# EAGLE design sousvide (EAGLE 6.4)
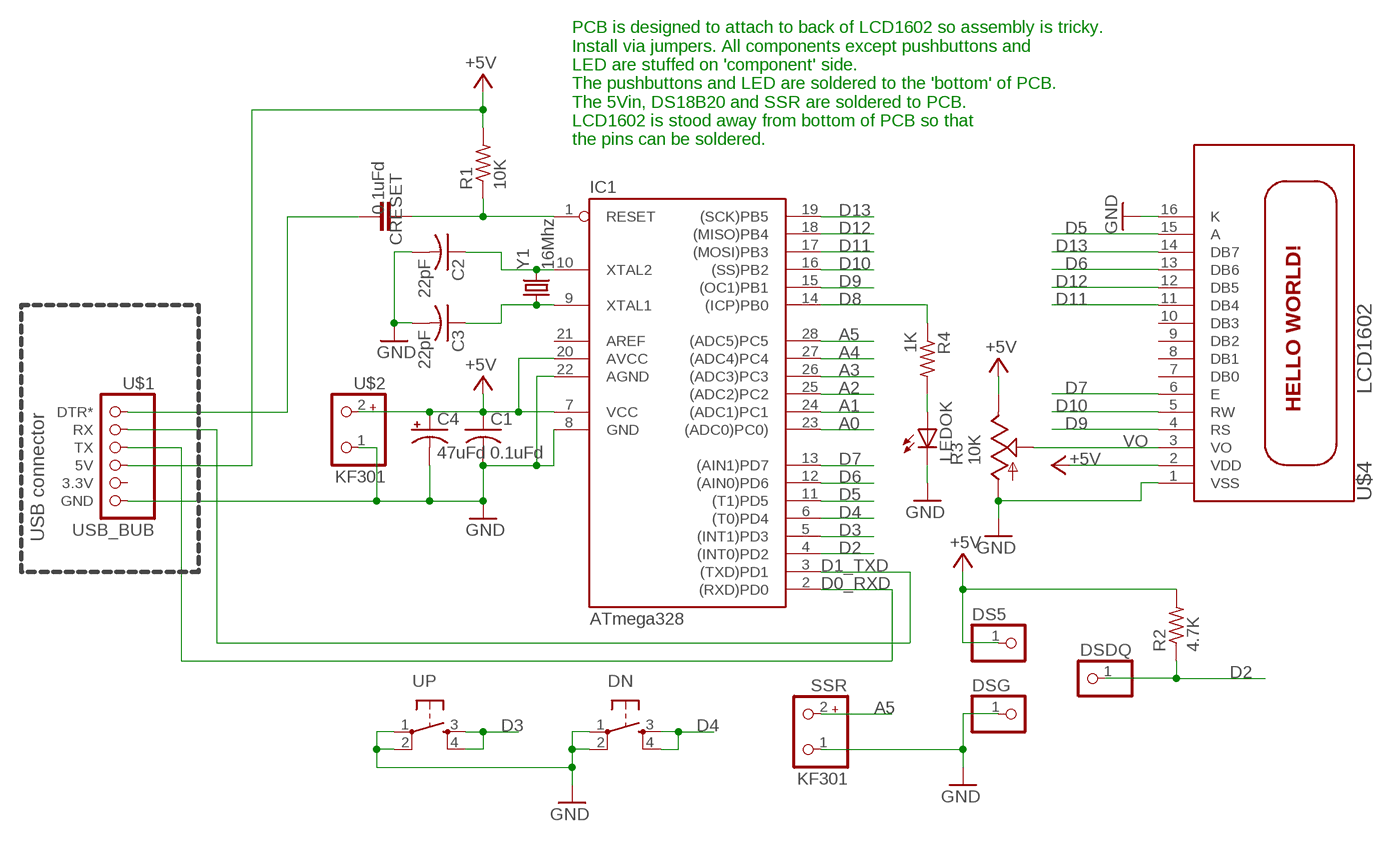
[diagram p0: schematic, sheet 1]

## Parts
C1  0.1uFd  C-US050-024X044  [C050-024X044]
C2  22pF  C-US025-024X044  [C025-024X044]
C3  22pF  C-US025-024X044  [C025-024X044]
C4  47uFd  CPOL-USE5-8.5  [E5-8,5]
CRESET  0.1uFd  C-EU050-045X075  [C050-045X075]
DN  TAC_SWITCHPTH  [TACTILE-PTH]
DS5  PINHD-1X1  [1X01]
DSDQ  PINHD-1X1  [1X01]
DSG  PINHD-1X1  [1X01]
IC1  ATmega328  AT90S4433P  [DIL28-3]
LEDOK  LED5MM  [LED5MM]
R1  10K  R-US_0207/2V  [0207/2V]
R2  4.7K  R-US_0204/7  [0204/7]
R3  10K  TRIM_US-B64Y  [B64Y]
R4  1K  R-US_0207/7  [0207/7]
SSR  KF301  [KF301]
U$1  USB_BUB  [USB_BUB]
U$2  KF301  [KF301]
U$4  LCD1602  [LCD1602]
UP  TAC_SWITCHPTH  [TACTILE-PTH]
Y1  16Mhz  CRYSTALHC49US  [HC49US]

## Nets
+5V [power]: C1.1 C4.+ DS5.1 IC1.7(VCC) IC1.20(AVCC) R1.2 R2.2 R3.E U$1.5V U$2.2 U$4.2(VDD)
A0: IC1.23((ADC0)PC0))
A1: IC1.24((ADC1)PC1)
A2: IC1.25((ADC2)PC2)
A3: IC1.26((ADC3)PC3)
A4: IC1.27((ADC4)PC4)
A5: IC1.28((ADC5)PC5) SSR.2
D0_RXD: IC1.2((RXD)PD0) U$1.TX
D1_TXD: IC1.3((TXD)PD1) U$1.RX
D2: DSDQ.1 IC1.4((INT0)PD2) R2.1
D3: IC1.5((INT1)PD3) UP.3 UP.4
D4: DN.3 DN.4 IC1.6((T0)PD4)
D5: IC1.11((T1)PD5) U$4.15(A)
D6: IC1.12((AIN0)PD6) U$4.13(DB6)
D7: IC1.13((AIN1)PD7) U$4.6(E)
D8: IC1.14((ICP)PB0) R4.1
D9: IC1.15((OC1)PB1) U$4.4(RS)
D10: IC1.16((SS)PB2) U$4.5(RW)
D11: IC1.17((MOSI)PB3) U$4.11(DB4)
D12: IC1.18((MISO)PB4) U$4.12(DB5)
D13: IC1.19((SCK)PB5) U$4.14(DB7)
GND [power]: C1.2 C2.2 C3.2 C4.- DN.1 DN.2 DSG.1 IC1.8(GND) IC1.22(AGND) LEDOK.K(C) R3.A SSR.1 U$1.GND U$2.1 U$4.1(VSS) U$4.16(K) UP.1 UP.2
N$1: LEDOK.A R4.2
N$6: C3.1 IC1.9(XTAL1) Y1.1
N$7: C2.1 IC1.10(XTAL2) Y1.2
N$8: CRESET.1 U$1.DTR*
RESET: CRESET.2 IC1.1(RESET) R1.1
VO: R3.S U$4.3(VO)
Unconnected: IC1.21(AREF) U$1.3.3V U$4.7(DB0) U$4.8(DB1) U$4.9(DB2) U$4.10(DB3)

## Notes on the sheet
- PCB is designed to attach to back of LCD1602 so assembly is tricky.
  Install via jumpers. All components except pushbuttons and
  LED are stuffed on 'component' side.
  The pushbuttons and LED are soldered to the 'bottom' of PCB. 
  The 5Vin, DS18B20 and SSR are soldered to PCB.
  LCD1602 is stood away from bottom of PCB so that
  the pins can be soldered.
- USB connector

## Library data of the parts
C1-C3 = MTS:C-US: CAPACITOR, American symbol
C4 = rcl:CPOL-US: POLARIZED CAPACITOR, American symbol
CRESET = my-rcl:C-EU: CAPACITOR, European symbol
DN UP = SparkFun:TAC_SWITCH: Momentary Switch Button commonly used for reset or general input. Spark Fun Electronics SKU : COM-00097
DS5 DSDQ DSG = pinhead:PINHD-1X1: PIN HEADER
IC1 = atmel:AT90S4433: MICROCONTROLLER 4 Kbytes FLASH 128 bytes SRAM 256 bytes EEPROM UART 6-channel 10 bit ADC
LEDOK = SparkFun:LED: LEDs
R1 R2 R4 = MTS:R-US_: RESISTOR, American symbol
R3 = pot:TRIM_US-: POTENTIOMETER
SSR U$2 = MTS_Custom:KF301
U$1 = MTS:USB_BUB
U$4 = MTS_Custom:LCD1602
Y1 = MTS:CRYSTAL: Crystals

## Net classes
0 default: width 0.4 mm, clearance 0.3 mm
1 power: width 0.6 mm, clearance 0.3 mm

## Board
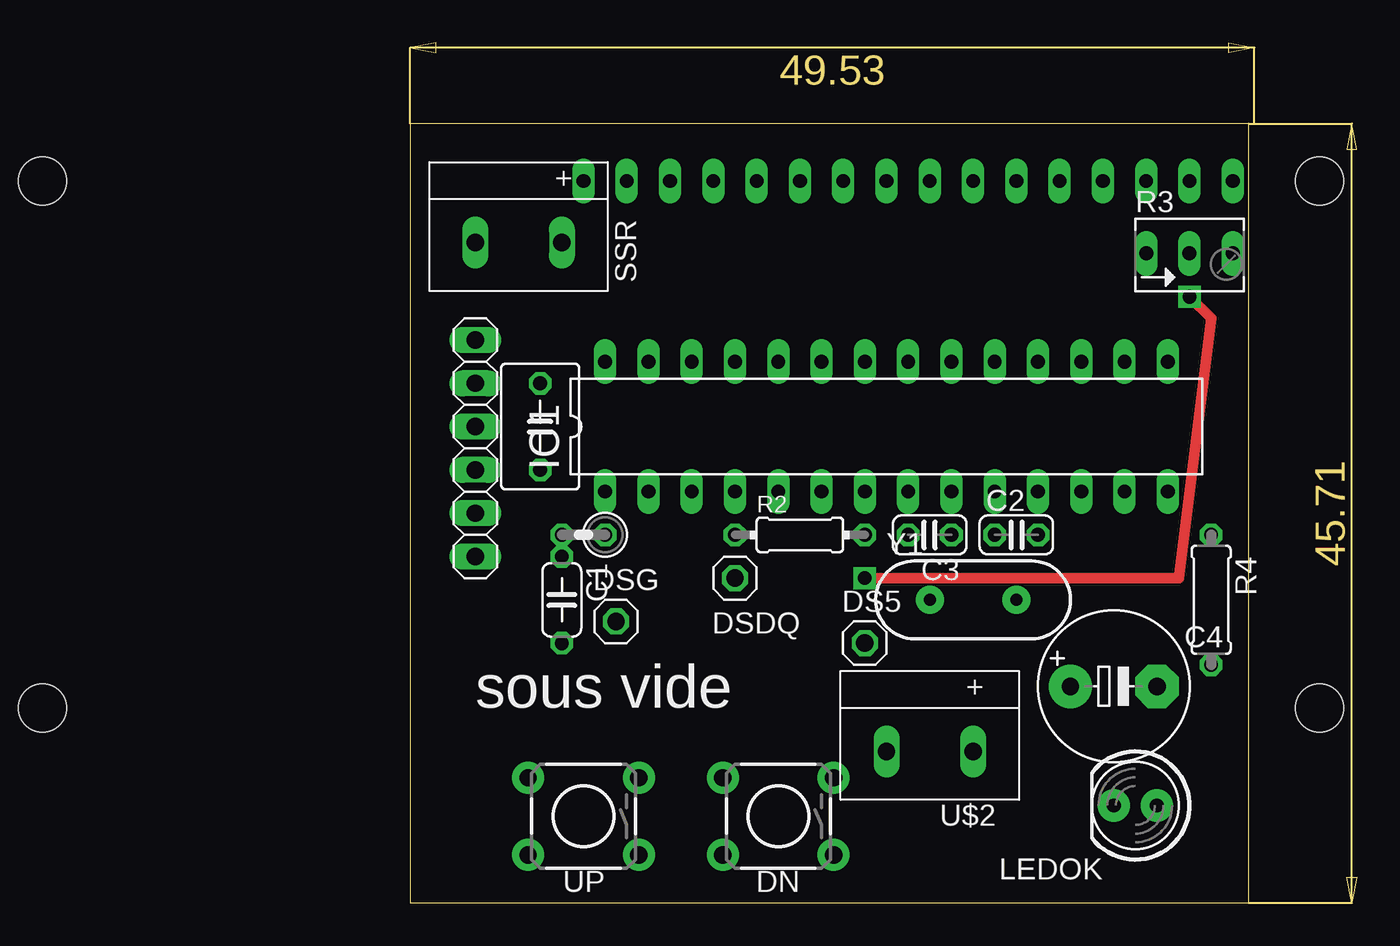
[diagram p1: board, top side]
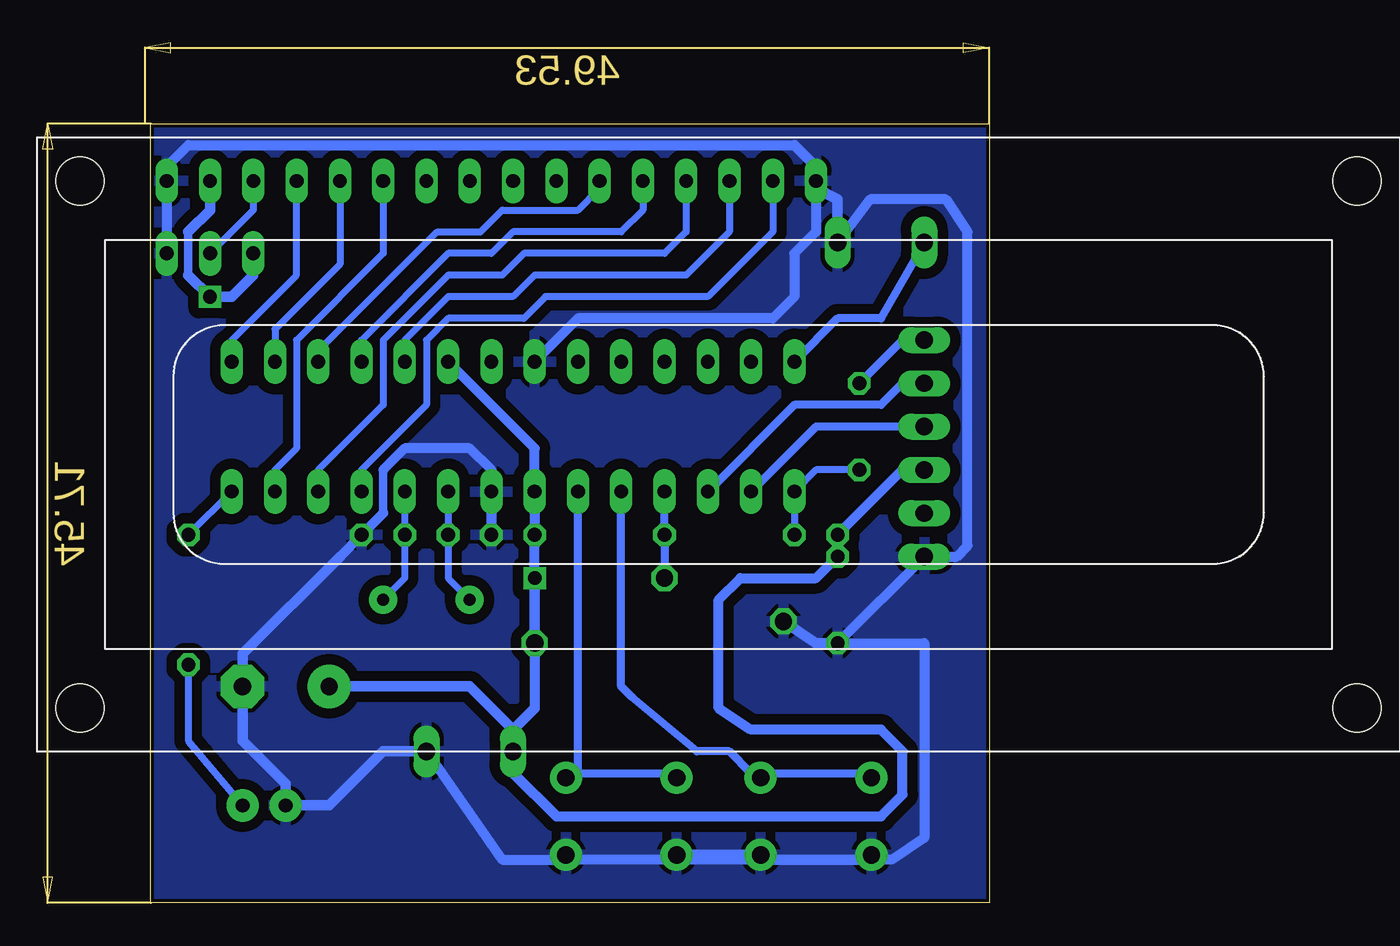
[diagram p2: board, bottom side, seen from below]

Size 55.54 x 50.46 mm. Coordinates in mm from the lower left corner, seen from the top.
Outline: 0,0 49.2,0 49.2,45.71 0,45.71 0,0
Copper layers (1*16): Top 0.035mm / dielectric 1.5mm / Bottom 0.035mm
Design rules "MTS": minimum track width 18mil, minimum drill 12mil, track to track 24mil, track to pad 24mil, pad to pad 6mil, via to via 6mil, smd to smd 0mil, copper to edge 8mil, drill to drill 10mil, minimum pad ring 10mil, minimum via ring 10mil, stop-mask expansion 2mil, vias tented up to drill 25mil, thermal gap 10mil

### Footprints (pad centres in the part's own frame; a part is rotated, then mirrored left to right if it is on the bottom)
C050-024X044 = drill 0.813 octagon: 1 -2.54,0; 2 2.54,0
C025-024X044 = drill 0.813 octagon: 1 -1.27,0; 2 1.27,0
E5-8,5 = drill 1.016 pad 2.54: + -2.54,0 | drill 1.016 pad 2.54 octagon: - 2.54,0
C050-045X075 = drill 0.813 octagon: 1 -2.54,0; 2 2.54,0
TACTILE-PTH = drill 1.016 pad 1.88: 1 -3.251,2.261; 2 3.251,2.261; 3 -3.251,-2.261; 4 3.251,-2.261
1X01 = drill 1.016 octagon: 1 0,0
DIL28-3 = drill 0.813 long: 1 -16.51,-3.81; 2 -13.97,-3.81; 3 -11.43,-3.81; 4 -8.89,-3.81; 5 -6.35,-3.81; 6 -3.81,-3.81; 7 -1.27,-3.81; 8 1.27,-3.81; 9 3.81,-3.81; 10 6.35,-3.81; 11 8.89,-3.81; 12 11.43,-3.81; 13 13.97,-3.81; 14 16.51,-3.81; 15 16.51,3.81; 16 13.97,3.81; 17 11.43,3.81; 18 8.89,3.81; 19 6.35,3.81; 20 3.81,3.81; 21 1.27,3.81; 22 -1.27,3.81; 23 -3.81,3.81; 24 -6.35,3.81; 25 -8.89,3.81; 26 -11.43,3.81; 27 -13.97,3.81; 28 -16.51,3.81
LED5MM = drill 0.813 pad 1.88: A -1.27,0; K 1.27,0
0207/2V = drill 0.813 octagon: 1 -1.27,0; 2 1.27,0
0204/7 = drill 0.813 octagon: 1 -3.81,0; 2 3.81,0
B64Y = drill 0.813 long: A 2.54,0; E -2.54,0; S 0,0
0207/7 = drill 0.813 octagon: 1 -3.81,0; 2 3.81,0
KF301 = drill 1.016 long: 1 -2.54,0; 2 2.54,0
USB_BUB = drill 1.016 long: 3.3V -3.81,0; 5V -1.27,0; DTR* 6.35,0; GND -6.35,0; RX 3.81,0; TX 1.27,0
LCD1602 = drill 0.8 long: 1 7.62,33.46; 2 10.16,33.46; 3 12.7,33.46; 4 15.24,33.46; 5 17.78,33.46; 6 20.32,33.46; 7 22.86,33.46; 8 25.4,33.46; 9 27.94,33.46; 10 30.48,33.46; 11 33.02,33.46; 12 35.56,33.46; 13 38.1,33.46; 14 40.64,33.46; 15 43.18,33.46; 16 45.72,33.46 | hole 2.8: 2.54,2.54; 2.54,33.46; 77.46,33.46; 77.46,2.54
HC49US = drill 0.7 pad 1.651: 1 -2.54,0; 2 2.54,0

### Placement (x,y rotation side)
C1  8.89,17.78 270 top
C2  35.56,21.59 0 top
C3  30.48,21.59 180 top
C4  41.27,12.7 0 top
CRESET  7.62,27.94 270 top
DN  21.59,5.08 180 top
DS5  26.67,15.24 0 top
DSDQ  19.05,19.05 0 top
DSG  12.06,16.51 0 top
IC1  27.94,27.94 0 top
LEDOK  42.55,5.71 180 top
R1  10.16,21.59 180 top
R2  22.86,21.59 0 top
R3  45.72,38.1 0 top
R4  46.99,17.78 270 top
SSR  6.35,38.73 180 top
U$1  3.81,26.67 90 top
U$2  30.48,8.89 180 top
U$4  55.88,8.89 0 bottom
UP  10.16,5.08 180 top
Y1  33.02,17.78 0 top

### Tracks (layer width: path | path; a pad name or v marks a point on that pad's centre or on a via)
+5V  (via drill 0.8)
  Top 0.61: v45.72,35.56 46.99,34.29 45.09,19.05 v26.67,19.05
  Bottom 0.508: 46.99,39.37 46.99,36.83
  Bottom 0.6: U$1.5V 5.08,25.4 R1.2 C1.1 10.16,19.05 14.61,19.05 15.88,17.78 15.88,11.43 13.97,10.16 6.35,10.16 5.08,8.89 5.08,6.35 6.35,5.08 25.4,5.08 | IC1.20 26.67,26.67 IC1.7 R2.2 v26.67,19.05 | DS5.1 26.67,11.43
  Bottom 0.61: U$4.2 45.72,40.64 46.99,39.37 | 46.99,36.83 v45.72,35.56 44.45,35.56 43.18,36.83 R3.E | v26.67,19.05 DS5.1 | 27.94,10.16 26.67,11.43 | C4.+ 30.48,12.7 27.94,10.16 | 27.94,10.16 U$2.2 27.94,7.62 25.4,5.08
A5
  Bottom 0.457: IC1.28 8.89,34.29 6.35,34.29 SSR.2
D0_RXD
  Bottom 0.457: IC1.2 10.16,27.94 U$1.TX
D1_TXD
  Bottom 0.457: IC1.3 11.43,29.21 6.35,29.21 5.08,30.48 U$1.RX
D2
  Bottom 0.457: IC1.4 R2.1 DSDQ.1
D3
  Bottom 0.457: IC1.5 21.59,12.7 20.95,12.06 17.14,8.89 15.24,8.89 13.97,7.62 UP.3 12.7,7.62 7.62,7.62 UP.4
D4
  Bottom 0.457: 24.13,7.62 IC1.6 | 24.13,7.62 19.05,7.62 DN.4 | 24.13,7.62 DN.3
D5
  Bottom 0.406: U$4.15 12.7,39.37 16.51,35.56 26.04,35.56 27.3,34.29 31.75,34.29 33.02,33.02 33.02,29.21 36.83,25.4 IC1.11
D6
  Bottom 0.406: U$4.13 17.78,39.37 19.05,38.1 27.3,38.1 28.57,36.83 31.75,36.83 35.56,33.02 35.56,29.21 39.37,25.4 IC1.12
D7
  Bottom 0.406: U$4.6 35.56,38.1 40.64,33.02 40.64,26.67 41.91,25.4 IC1.13
D8
  Bottom 0.406: IC1.14 R4.1
D9
  Bottom 0.406: IC1.15 44.45,33.02 40.64,36.83 U$4.4
D10
  Bottom 0.406: U$4.5 38.1,37.47 41.91,33.66 IC1.16
D11
  Bottom 0.406: IC1.17 39.37,32.38 32.38,39.37 29.84,39.37 28.57,40.64 24.13,40.64 22.86,41.91 U$4.11
D12
  Bottom 0.406: U$4.12 20.32,40.64 21.59,39.37 27.94,39.37 29.21,38.1 31.75,38.1 36.83,33.02 IC1.18
D13
  Bottom 0.406: U$4.14 15.24,39.37 17.78,36.83 26.67,36.83 27.94,35.56 31.75,35.56 34.29,33.02 IC1.19
GND
  Bottom 0.508: 35.56,25.4 35.56,22.86
  Bottom 0.6: 35.56,22.86 C2.2 38.1,20.32 | 35.56,25.4 34.29,26.67 30.48,26.67 29.21,25.4 IC1.8 C3.2 | IC1.22 24.13,34.29 12.7,34.29 11.43,35.56 11.43,38.1 10.16,39.37 10.16,41.91 | DN.2 19.05,2.54 24.13,2.54 DN.1 24.77,2.54 | 11.43,44.45 46.99,44.45 48.26,43.18 U$4.1 R3.A | 24.77,2.54 28.57,2.54 U$2.1 | SSR.1 6.99,41.27 2.54,41.27 1.27,39.37 1.27,20.95 1.91,20.32 U$1.GND C1.2 3.81,15.24 3.81,3.81 5.71,2.54 24.77,2.54 | UP.2 7.62,2.54 12.7,2.54 UP.1
  Bottom 0.61: C1.2 10.16,15.24 DSG.1 | SSR.1 8.89,41.27 10.16,41.91 U$4.16 10.16,43.18 11.43,44.45 | 38.1,20.32 43.81,14.61 C4.- 43.81,9.53 41.27,6.99 LEDOK.K 38.73,5.71 35.56,8.89 U$2.1 | DN.2 UP.1
  pour Bottom: 0,0 49.53,0 49.53,45.72 0,45.72
N$1
  Bottom 0.406: R4.2 46.99,9.53 LEDOK.A
N$6
  Bottom 0.4: IC1.9 C3.1 31.75,19.05 Y1.1
N$7
  Bottom 0.4: IC1.10 C2.1 34.29,19.05 Y1.2
N$8
  Bottom 0.457: CRESET.1 5.08,33.02 U$1.DTR*
RESET
  Bottom 0.406: CRESET.2 10.16,25.4 IC1.1 R1.1
VO
  Bottom 0.406: U$4.3 43.18,40.64 R3.S

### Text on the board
tNames: sous vide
